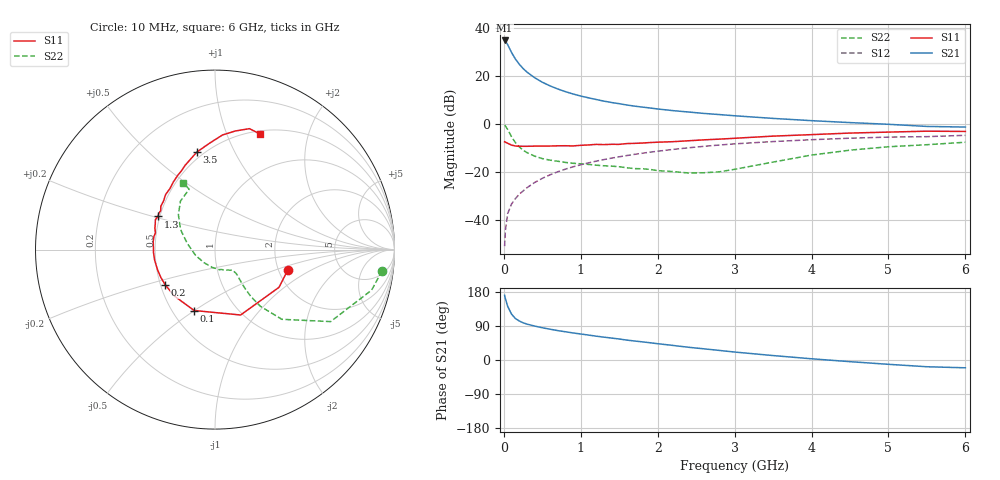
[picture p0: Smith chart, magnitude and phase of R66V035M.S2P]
! SIEMENS Small Signal Semiconductors
! BFR193
! Si NPN RF Bipolar Junction Transistor in SOT23
! VCE = 6 V  IC = 35 mA
! Common Emitter S-Parameters:  May  1996
# GHz  S  MA  R  50
!  f  S11  S21  S12  S22
! GHz  MAG  ANG  MAG  ANG  MAG  ANG  MAG  ANG
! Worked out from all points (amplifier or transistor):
!   36 points, 10 MHz to 6 GHz, reference 50 ohm
!   highest |S21| = 34.8 dB at 10 MHz (marker M1)
!   |S21| within 3 dB of that: start of sweep to 68.7 MHz
!   unconditionally stable (mu >= 1): 483.5 MHz to 1.967 GHz
!   at 250 MHz: K = 0.91, MSG = 25.5 dB, |S12| = -28.0 dB
!   at 1.4 GHz: K = 1.02, MAG = 10.7 dB, |S12| = -14.3 dB
!   at 6 GHz: K = 0.95, MSG = 1.7 dB, |S12| = -4.8 dB
!   S11 on the Smith chart (normalised r, x): 10 MHz: 2.25, -0.62; 100 MHz: 0.64, -0.50; 200 MHz: 0.53, -0.24; 1.3 GHz: 0.49, +0.21; 3.5 GHz: 0.46, +0.72; 6 GHz: 0.53, +1.32
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0.01  0.4213 -15.6  54.65 170.7  0.0028 83.6  0.9386 -7.2
0.02  0.414 -30.5  53.16 162.1  0.0059 80.0  0.9013 -14.5
0.05  0.3913 -68.6  44.45 141.5  0.0134 71.3  0.7591 -31.9
0.1  0.3588 -108.9  30.66 121.1  0.0212 66.9  0.5382 -46.2
0.15  0.3437 -131.3  22.45 109.5  0.0274 66.7  0.4051 -51.3
0.2  0.3398 -144.7  17.52 103.0  0.0339 68.5  0.3301 -52.6
0.25  0.3392 -153.1  14.2 98.2  0.0396 69.4  0.2816 -52.4
0.3  0.3392 -160.3  12.01 94.7  0.0463 71.1  0.251 -51.8
0.4  0.3416 -170.2  9.148 89.6  0.0595 71.8  0.2115 -50.2
0.5  0.343 -177.3  7.351 85.1  0.0728 72.0  0.1877 -48.8
0.6  0.3432 178.0  6.175 81.3  0.0861 71.8  0.1743 -48.5
0.7  0.347 172.7  5.326 77.6  0.0996 71.3  0.1654 -48.9
0.8  0.3482 168.2  4.676 74.5  0.1131 70.4  0.1563 -49.4
0.9  0.3448 164.3  4.179 71.4  0.1267 69.5  0.15 -50.0
1.1  0.3614 157.1  3.475 65.8  0.1529 67.4  0.1421 -54.1
1.3  0.3678 149.9  2.969 60.3  0.1792 64.7  0.1331 -58.3
1.7  0.3905 138.7  2.332 50.1  0.2303 59.4  0.1161 -72.1
2.2  0.4232 126.3  1.878 38.4  0.292 52.1  0.1006 -98.7
3.5  0.5524 100.6  1.294 11.7  0.4257 32.1  0.159 167.2
4.5  0.6397 86.3  1.058 -4.4  0.5003 18.1  0.2816 136.4
5.5  0.7006 74.1  0.88 -17.8  0.5387 4.3  0.3658 113.2
6  0.6917 68.8  0.854 -20.6  0.5743 0.4  0.4117 115.4
